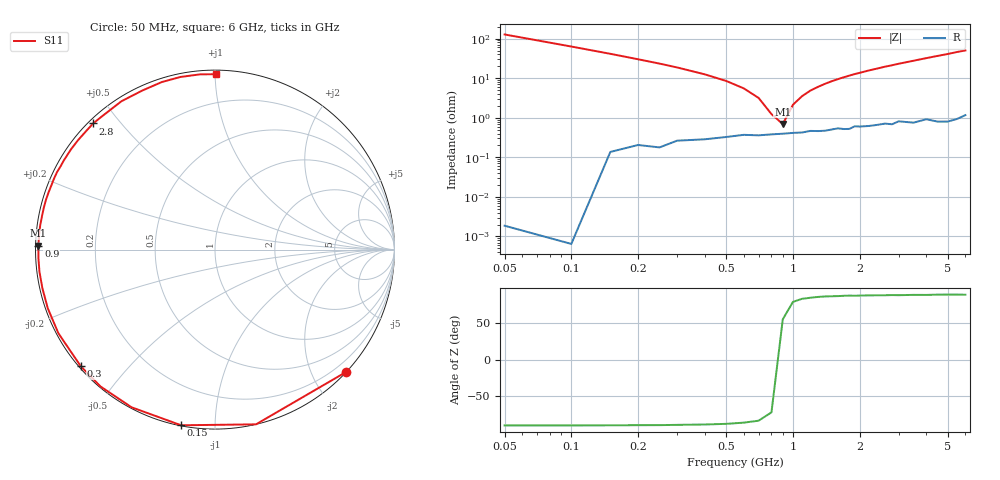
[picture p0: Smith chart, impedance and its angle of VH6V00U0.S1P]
! Infineon Technologies  Discrete & RF Semiconductors
! BB 814
! Si Tuning Diode in SOT23
! VR = 6 V
! S-Parameters:  July  1999
# GHz  S  MA  R  50
!  f  S11
! GHz  MAG  ANG
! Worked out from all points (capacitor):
!   34 points, 50 MHz to 6 GHz, reference 50 ohm
!   read as one part to ground: C = 24.9 pF near 50 MHz
!   lowest |Z| = 691 mohm at 900 MHz (marker M1)
!   series resonance near 867.5 MHz, so ESL is about 1.4 nH
!   S11 on the Smith chart (normalised r, x): 50 MHz: 0.00, -2.55; 150 MHz: 0.00, -0.83; 300 MHz: 0.01, -0.37; 900 MHz: 0.01, +0.01; 2.8 GHz: 0.01, +0.42; 6 GHz: 0.02, +1.00
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0.05  1 -42.9
0.1  1 -76.8
0.15  0.9968 -100.9
0.2  0.994 -117.9
0.25  0.9942 -129.9
0.3  0.9908 -139.0
0.4  0.9893 -151.9
0.5  0.9874 -160.7
0.6  0.9855 -167.4
0.7  0.9858 -172.8
0.8  0.9849 -177.3
0.9  0.9843 178.7
1  0.9836 175.2
1.2  0.9817 168.9
1.4  0.9817 163.5
1.6  0.9794 158.5
1.9  0.9774 151.5
2.2  0.9777 145.2
2.4  0.9767 141.4
2.6  0.9756 137.4
2.8  0.977 134.0
3  0.9736 130.3
3.5  0.9772 122.2
4  0.9744 114.5
4.5  0.9794 107.6
5  0.9809 101.4
5.5  0.98 94.9
6  0.9771 89.7
